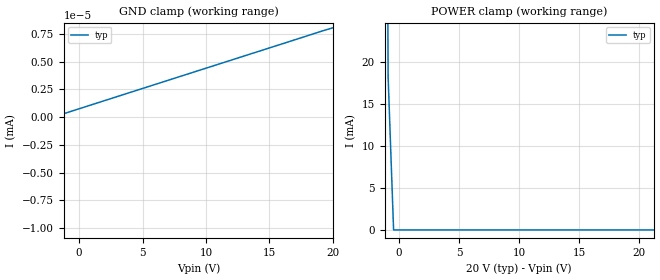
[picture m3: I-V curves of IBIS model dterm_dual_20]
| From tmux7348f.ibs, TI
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| dterm_dual_20
[Model]   dterm_dual_20
Model_type   Terminator
|   typ   min   max
C_comp   1.008417e-11   NA   NA
[Voltage Range]   20   NA   NA
[Temperature Range]   27   NA   NA
[Power Clamp Reference]   20   NA   NA
[GND Clamp Reference]   0   NA   NA
[GND Clamp]
|   Voltage   I(typ)   I(min)   I(max)
-25V      -1.414A    NA         NA
-20V      -5.041uA   NA         NA
-19.55V   -6.406nA   NA         NA
20V       8.043nA    NA         NA
[POWER Clamp]
|   Voltage   I(typ)   I(min)   I(max)
-5V       1.414A     NA         NA
-1.364V   155.3mA    NA         NA
-909.1mV  18.23mA    NA         NA
-454.5mV  68.57nA    NA         NA
40V       -5.036uA   NA         NA
